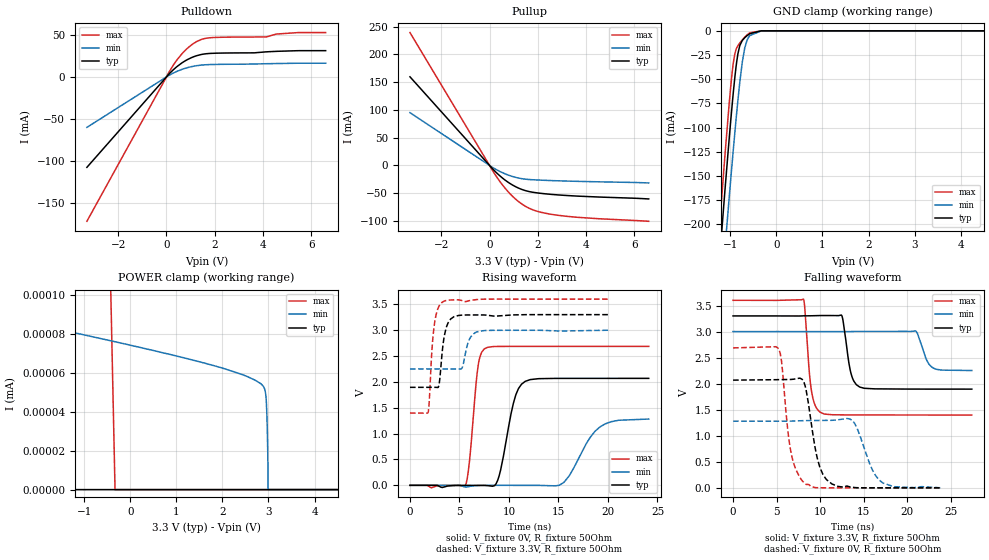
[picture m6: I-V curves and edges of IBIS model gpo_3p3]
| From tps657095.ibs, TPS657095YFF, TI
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|   gpo_3p3 Model
[Model]   gpo_3p3
Model_type   3-state
Polarity   Non-Inverting
Vmeas = 1.65
Vref = 0
Cref = 2pF
Rref = 200
|   typ   min   max
|   (nom PVT)   (fast PVT)   (slow PVT)
C_comp   7.098e-12   6.950e-12   7.329e-12
| Where nom  PVT is Nominal Process, 3.3V, 27C
|   Fast PVT is Strong Process,  3.6V, -40C
|   Slow PVT is Weak Process,   3V, 125C
[Voltage Range]   3.3   3   3.6
|Junction Temperature
[Temperature Range]   27   125   -40
[Pullup Reference]   3.3   3   3.6
[Pulldown Reference]   0   0   0
[Power Clamp Reference]   3.3   3   3.6
[GND Clamp Reference]   0   0   0
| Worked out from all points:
|   slope of the pulldown table from 0 to 0.495 V, typ, clamps not added: 36.3 ohm
|   slope of the pullup table from 0 to 0.495 V, typ, clamps not added: 23.3 ohm
|   GND clamp passes 1 mA (typ) near -0.41 V on its own axis
|   POWER clamp passes 1 mA (typ) near -2.44 V on its own axis
|   falling waveform, V_fixture 3.3V, R_fixture 50Ohm: 20-80 % time 787ps typ, 988ps min, 667ps max; typ from 3.3 V to 1.9 V
|   rising waveform, V_fixture 0V, R_fixture 50Ohm: 20-80 % time 1.27ns typ, 2.31ns min, 728ps max; typ from 0 V to 2.07 V
|   rising waveform, V_fixture 3.3V, R_fixture 50Ohm: 20-80 % time 550ps typ, 631ps min, 494ps max; typ from 1.9 V to 3.3 V
|   falling waveform, V_fixture 0V, R_fixture 50Ohm: 20-80 % time 1.31ns typ, 1.77ns min, 1.12ns max; typ from 2.07 V to 0 V
[Pulldown]
|   Voltage   I(typ)   I(min)   I(max)
-3.3V     -107.5mA   -59.99mA   -171.7mA
147mV     4.705mA    2.543mA    7.741mA
408mV     11.67mA    6.303mA    19.2mA
645.6mV   16.8mA     9.043mA    27.68mA
1.031V    22.9mA     12.23mA    37.95mA
1.44V     26.69mA    14.08mA    44.54mA
1.791V    27.95mA    14.71mA    46.6mA
3.633V    28.66mA    15.4mA     47.51mA
4.148V    29.89mA    15.74mA    47.67mA
4.559V    30.46mA    15.93mA    51.03mA
5.491V    31.25mA    16.32mA    52.79mA
6.6V      31.25mA    16.32mA    52.8mA
[GND Clamp]
|   Voltage   I(typ)   I(min)   I(max)
-3.3V     -1.612A    -1.624A    -1.62A
-1.296V   -274.8mA   -332.7mA   -241.5mA
-1.136V   -176.7mA   -237.1mA   -140.6mA
-1.107V   -159.1mA   -219.8mA   -122.7mA
-1.025V   -111.5mA   -172.4mA   -75.2mA
-954mV    -73.14mA   -133mA     -40.37mA
-902.4mV  -48.24mA   -105.3mA   -23.88mA
-834.9mV  -23.62mA   -71.52mA   -15.34mA
-741mV    -9.998mA   -32.55mA   -9.379mA
-687mV    -7.094mA   -17.64mA   -6.531mA
-576mV    -2.925mA   -4.891mA   -2.025mA
6.6V      0A         0A         0A
[Pullup]
|   Voltage   I(typ)   I(min)   I(max)
-3.3V     159.6mA    95.02mA    239.3mA
153mV     -7.348mA   -4.284mA   -11.23mA
423mV     -18.57mA   -10.74mA   -28.61mA
660mV     -26.92mA   -15.43mA   -41.82mA
933.6mV   -34.84mA   -19.7mA    -54.76mA
1.168V    -40.19mA   -22.42mA   -63.92mA
1.449V    -44.89mA   -24.55mA   -72.59mA
1.773V    -48.17mA   -25.75mA   -79.6mA
2.577V    -52.21mA   -27.3mA    -88.19mA
3.633V    -55.23mA   -28.67mA   -93.39mA
6.6V      -60.34mA   -31.55mA   -100.6mA
[POWER Clamp]
|   Voltage   I(typ)   I(min)   I(max)
-3.3V     2.469mA    761uA      6.841mA
-2.193V   33.73uA    156.2nA    2.462mA
-1.996V   112.5nA    84.97nA    338uA
-1.968V   43.33nA    84.69nA    198.3uA
-1.936V   14.5nA     84.47nA    95.43uA
-1.885V   0A         84.18nA    23.56uA
-330mV    0A         76.03nA    0A
2.844V    0A         54.24nA    0A
2.949V    0A         46.73nA    0A
2.978V    0A         26.66nA    0A
2.991V    0A         0A         0A
6.6V      0A         0A         0A
[Ramp]
R_load = 50
|   typ   min   max
dV/dt_r   1.24073/1.25061e-09   0.768084/2.28638e-09   1.61196/7.2614e-10
dV/dt_f   0.843179/7.83189e-10   0.449747/9.84574e-10   1.32104/6.64491e-10
[Falling Waveform]
V_fixture = 3.3V
V_fixture_min = 3V
V_fixture_max = 3.6V
R_fixture = 50Ohm
|   Time   V(typ)   V(min)   V(max)
0s        3.3V       3V         3.6V
8.083ns   3.302V     3V         3.623V
8.978ns   3.303V     3V         1.886V
9.997ns   3.307V     3V         1.452V
12.51ns   3.296V     2.999V     1.401V
13.53ns   2.206V     3V         1.4V
14.5ns    1.939V     3.001V     1.4V
20.94ns   1.896V     3.011V     1.398V
22.71ns   1.895V     2.332V     1.398V
27.41ns   1.895V     2.252V     1.398V
[Rising Waveform]
V_fixture = 0V
V_fixture_min = 0V
V_fixture_max = 0V
R_fixture = 50Ohm
|   Time   V(typ)   V(min)   V(max)
0s        172.8pV    7.896nV    97.26pV
5.586ns   -200.8uV   -30.6mV    -6.13mV
6.895ns   -1.519mV   -3.161mV   2.326V
7.525ns   -1.902mV   -825.5uV   2.64V
8.865ns   98.41mV    -61.66uV   2.685V
10.45ns   1.589V     -494.4uV   2.686V
11.65ns   2.011V     -750.6uV   2.686V
15.55ns   2.068V     56.97mV    2.687V
19.69ns   2.068V     1.185V     2.687V
24.12ns   2.068V     1.282V     2.687V
[Rising Waveform]
V_fixture = 3.3V
V_fixture_min = 3V
V_fixture_max = 3.6V
R_fixture = 50Ohm
|   Time   V(typ)   V(min)   V(max)
0s        1.895V     2.25V      1.398V
1.838ns   1.895V     2.25V      1.412V
2.448ns   1.895V     2.25V      3.087V
2.933ns   1.939V     2.25V      3.464V
3.342ns   2.727V     2.25V      3.55V
3.846ns   3.14V      2.25V      3.58V
5.184ns   3.289V     2.25V      3.576V
5.931ns   3.294V     2.793V     3.568V
6.967ns   3.294V     2.978V     3.596V
20.22ns   3.3V       3V         3.6V
[Falling Waveform]
V_fixture = 0V
V_fixture_min = 0V
V_fixture_max = 0V
R_fixture = 50Ohm
|   Time   V(typ)   V(min)   V(max)
0s        2.068V     1.28V      2.687V
5.247ns   2.077V     1.28V      2.671V
5.571ns   2.078V     1.28V      2.417V
6.637ns   2.081V     1.281V     693.1mV
8.391ns   1.873V     1.291V     66.09mV
9.654ns   578.5mV    1.294V     2.85mV
11.34ns   76.19mV    1.297V     975.6uV
13.91ns   6.809mV    1.249V     388uV
17.2ns    772.9uV    93.54mV    151.6uV
23.86ns   195.8uV    1.227mV    34.39uV
